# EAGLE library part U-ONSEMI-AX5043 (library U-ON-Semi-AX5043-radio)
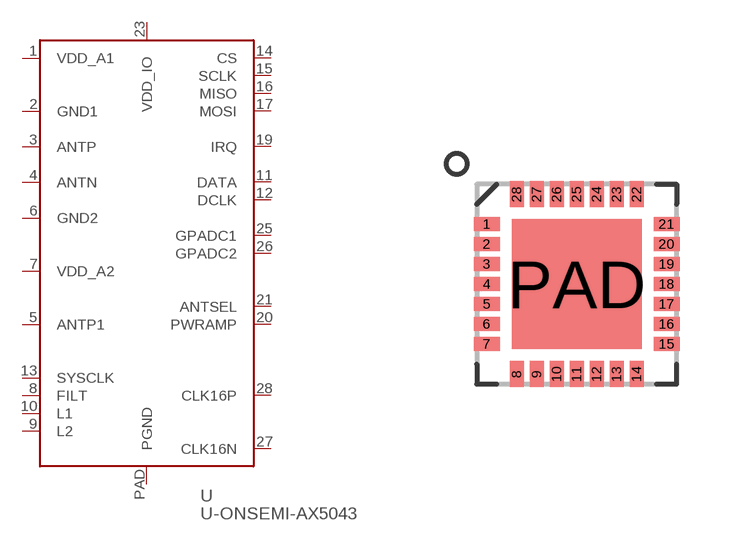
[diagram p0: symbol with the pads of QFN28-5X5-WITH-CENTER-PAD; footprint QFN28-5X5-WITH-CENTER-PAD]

Designator prefix U

## U-ONSEMI-AX5043  [QFN28-5X5-WITH-CENTER-PAD]
1  VDD_A1  pwr
2  GND1  pwr
3  ANTP
4  ANTN
5  ANTP1
6  GND2  pwr
7  VDD_A2  pwr
8  FILT  out
9  L2  in
10  L1  in
11  DATA
12  DCLK
13  SYSCLK
14  CS  in
15  SCLK  in
16  MISO  out
17  MOSI  in
19  IRQ
20  PWRAMP
21  ANTSEL
23  VDD_IO  pwr
25  GPADC1  in
26  GPADC2  in
27  CLK16N  pas
28  CLK16P  pas
PAD  PGND  pwr

## Footprint QFN28-5X5-WITH-CENTER-PAD (pad centres in mm)
smd 0.65 x 0.35: 1 -2.25,1.5; 2 -2.25,1; 3 -2.25,0.5; 4 -2.25,0; 5 -2.25,-0.5; 6 -2.25,-1; 7 -2.25,-1.5; 15 2.25,-1.5; 16 2.25,-1; 17 2.25,-0.5; 18 2.25,0; 19 2.25,0.5; 20 2.25,1; 21 2.25,1.5
smd 0.35 x 0.65: 8 -1.5,-2.25; 9 -1,-2.25; 10 -0.5,-2.25; 11 0,-2.25; 12 0.5,-2.25; 13 1,-2.25; 14 1.5,-2.25; 22 1.5,2.25; 23 1,2.25; 24 0.5,2.25; 25 0,2.25; 26 -0.5,2.25; 27 -1,2.25; 28 -1.5,2.25
smd 3.25 x 3.25: PAD 0,0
